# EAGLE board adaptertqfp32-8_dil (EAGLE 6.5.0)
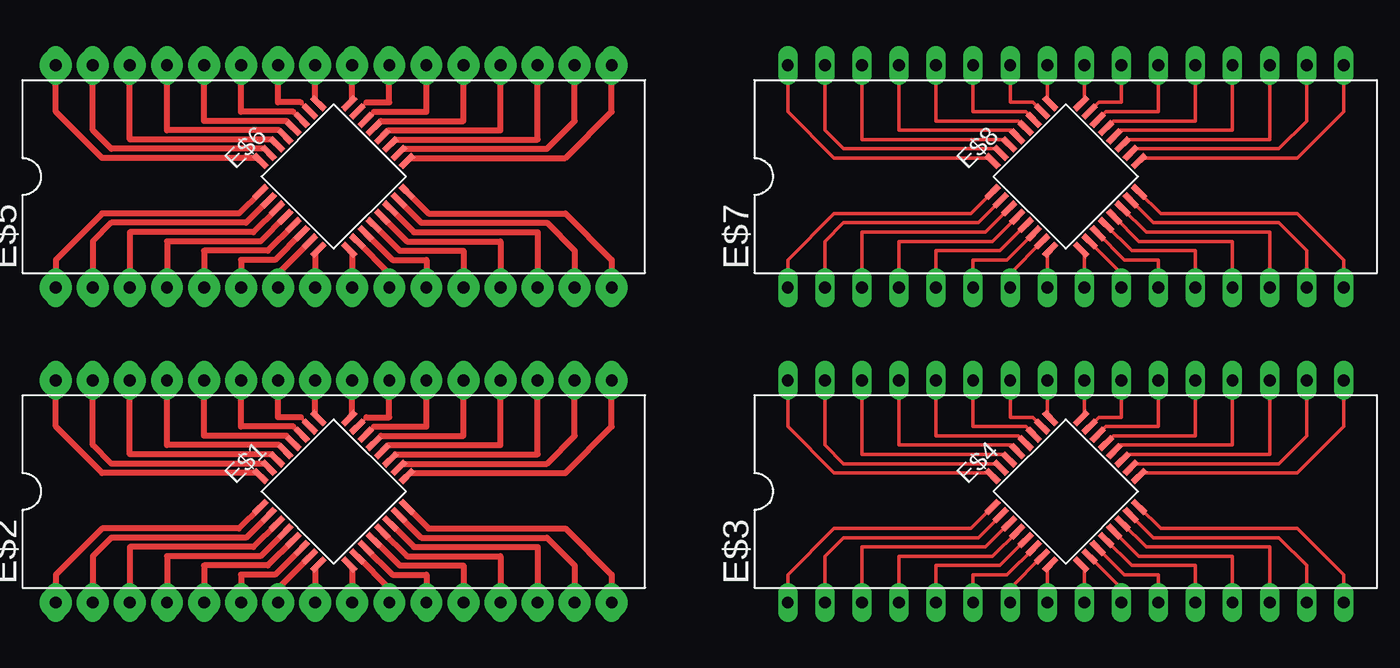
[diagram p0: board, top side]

No outline drawn. Coordinates in mm, seen from the top.
Copper layers (1*16): Top 0.035mm / dielectric 1.5mm / Bottom 0.035mm
Design rules "default": minimum track width 10mil, minimum drill 24mil, track to track 8mil, track to pad 8mil, pad to pad 8mil, via to via 8mil, smd to smd 8mil, copper to edge 40mil, drill to drill 8mil, minimum pad ring 10mil, minimum via ring 8mil, stop-mask expansion 4mil, vias tented up to drill 0mil, thermal gap 10mil

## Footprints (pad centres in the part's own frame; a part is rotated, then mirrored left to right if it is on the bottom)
LQFP32-7X7 = smd 1.2 x 0.4: 1 -4.3,2.8; 2 -4.3,2; 3 -4.3,1.2; 4 -4.3,0.4; 5 -4.3,-0.4; 6 -4.3,-1.2; 7 -4.3,-2; 8 -4.3,-2.8; 17 4.3,-2.8; 18 4.3,-2; 19 4.3,-1.2; 20 4.3,-0.4; 21 4.3,0.4; 22 4.3,1.2; 23 4.3,2; 24 4.3,2.8 | smd 0.4 x 1.2: 9 -2.8,-4.3; 10 -2,-4.3; 11 -1.2,-4.3; 12 -0.4,-4.3; 13 0.4,-4.3; 14 1.2,-4.3; 15 2,-4.3; 16 2.8,-4.3; 25 2.8,4.3; 26 2,4.3; 27 1.2,4.3; 28 0.4,4.3; 29 -0.4,4.3; 30 -1.2,4.3; 31 -2,4.3; 32 -2.8,4.3
DIL32 = drill 0.813 long: 1 -19.05,-7.62; 2 -16.51,-7.62; 3 -13.97,-7.62; 4 -11.43,-7.62; 5 -8.89,-7.62; 6 -6.35,-7.62; 7 -3.81,-7.62; 8 -1.27,-7.62; 9 1.27,-7.62; 10 3.81,-7.62; 11 6.35,-7.62; 12 8.89,-7.62; 13 11.43,-7.62; 14 13.97,-7.62; 15 16.51,-7.62; 16 19.05,-7.62; 17 19.05,7.62; 18 16.51,7.62; 19 13.97,7.62; 20 11.43,7.62; 21 8.89,7.62; 22 6.35,7.62; 23 3.81,7.62; 24 1.27,7.62; 25 -1.27,7.62; 26 -3.81,7.62; 27 -6.35,7.62; 28 -8.89,7.62; 29 -11.43,7.62; 30 -13.97,7.62; 31 -16.51,7.62; 32 -19.05,7.62

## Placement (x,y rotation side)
E$1  [LQFP32-7X7]  24.13,12.06 45 top
E$2  [DIL32]  24.13,12.06 0 top
E$3  [DIL32]  74.3,12.06 0 top
E$4  [LQFP32-7X7]  74.3,12.06 45 top
E$5  [DIL32]  24.13,33.66 0 top
E$6  [LQFP32-7X7]  24.13,33.66 45 top
E$7  [DIL32]  74.3,33.66 0 top
E$8  [LQFP32-7X7]  74.3,33.66 45 top

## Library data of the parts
E$1 E$4 E$6 E$8 = st-microelectronics
E$2 E$3 E$5 E$7 = atmel

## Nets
S$1: E$1.32 E$2.32
S$2: E$1.30 E$2.30
S$3: E$1.31 E$2.31
S$4: E$1.29 E$2.29
S$5: E$1.28 E$2.28
S$6: E$1.27 E$2.27
S$7: E$1.26 E$2.26
S$8: E$1.25 E$2.25
S$9: E$1.24 E$2.24
S$10: E$1.23 E$2.23
S$11: E$1.22 E$2.22
S$12: E$1.21 E$2.21
S$13: E$1.20 E$2.20
S$14: E$1.19 E$2.19
S$15: E$1.18 E$2.18
S$16: E$1.17 E$2.17
S$17: E$1.16 E$2.16
S$18: E$1.15 E$2.15
S$19: E$1.9 E$2.9
S$20: E$1.10 E$2.10
S$21: E$1.11 E$2.11
S$22: E$1.12 E$2.12
S$23: E$1.13 E$2.13
S$24: E$1.14 E$2.14
S$25: E$1.8 E$2.8
S$26: E$1.7 E$2.7
S$27: E$1.6 E$2.6
S$28: E$1.5 E$2.5
S$29: E$1.4 E$2.4
S$30: E$1.3 E$2.3
S$31: E$1.2 E$2.2
S$32: E$1.1 E$2.1
S$33: E$3.32 E$4.32
S$34: E$3.31 E$4.31
S$35: E$3.18 E$4.18
S$36: E$3.17 E$4.17
S$37: E$3.16 E$4.16
S$38: E$3.15 E$4.15
S$39: E$3.2 E$4.2
S$40: E$3.1 E$4.1
S$41: E$3.30 E$4.30
S$42: E$3.29 E$4.29
S$43: E$3.28 E$4.28
S$44: E$3.27 E$4.27
S$45: E$3.26 E$4.26
S$46: E$3.25 E$4.25
S$47: E$3.24 E$4.24
S$48: E$3.23 E$4.23
S$49: E$3.22 E$4.22
S$50: E$3.21 E$4.21
S$51: E$3.20 E$4.20
S$52: E$3.19 E$4.19
S$53: E$3.9 E$4.9
S$54: E$3.10 E$4.10
S$55: E$3.11 E$4.11
S$56: E$3.12 E$4.12
S$57: E$3.13 E$4.13
S$58: E$3.14 E$4.14
S$59: E$3.8 E$4.8
S$60: E$3.7 E$4.7
S$61: E$3.6 E$4.6
S$62: E$3.5 E$4.5
S$63: E$3.4 E$4.4
S$64: E$3.3 E$4.3
S$65: E$5.32 E$6.32
S$66: E$5.31 E$6.31
S$67: E$5.18 E$6.18
S$68: E$5.17 E$6.17
S$69: E$5.16 E$6.16
S$70: E$5.15 E$6.15
S$71: E$5.2 E$6.2
S$72: E$5.1 E$6.1
S$73: E$5.30 E$6.30
S$74: E$5.29 E$6.29
S$75: E$5.28 E$6.28
S$76: E$5.27 E$6.27
S$77: E$5.26 E$6.26
S$78: E$5.25 E$6.25
S$79: E$5.24 E$6.24
S$80: E$5.23 E$6.23
S$81: E$5.22 E$6.22
S$82: E$5.21 E$6.21
S$83: E$5.20 E$6.20
S$84: E$5.19 E$6.19
S$85: E$5.9 E$6.9
S$87: E$5.10 E$6.10
S$88: E$5.11 E$6.11
S$89: E$5.12 E$6.12
S$90: E$5.13 E$6.13
S$91: E$5.14 E$6.14
S$93: E$5.8 E$6.8
S$94: E$5.7 E$6.7
S$95: E$5.6 E$6.6
S$96: E$5.5 E$6.5
S$97: E$7.32 E$8.32
S$98: E$7.31 E$8.31
S$99: E$7.18 E$8.18
S$100: E$7.17 E$8.17
S$101: E$7.16 E$8.16
S$102: E$7.15 E$8.15
S$103: E$7.2 E$8.2
S$104: E$7.1 E$8.1
S$105: E$7.30 E$8.30
S$106: E$7.29 E$8.29
S$107: E$7.28 E$8.28
S$108: E$7.27 E$8.27
S$109: E$7.26 E$8.26
S$110: E$7.25 E$8.25
S$111: E$7.24 E$8.24
S$112: E$7.23 E$8.23
S$113: E$7.22 E$8.22
S$114: E$7.21 E$8.21
S$115: E$7.20 E$8.20
S$116: E$7.19 E$8.19
S$117: E$7.9 E$8.9
S$118: E$7.10 E$8.10
S$119: E$7.11 E$8.11
S$120: E$7.12 E$8.12
S$121: E$7.13 E$8.13
S$122: E$7.14 E$8.14
S$123: E$7.8 E$8.8
S$124: E$7.7 E$8.7
S$125: E$7.6 E$8.6
S$126: E$7.5 E$8.5
S$127: E$7.4 E$8.4
S$128: E$7.3 E$8.3
S$130: E$5.4 E$6.4
S$131: E$5.3 E$6.3

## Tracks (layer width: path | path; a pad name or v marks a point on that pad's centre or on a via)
S$1
  Top 0.254: E$1.32 18.9,13.34
  Top 0.406: E$2.32 5.08,16.51 8.26,13.34 18.9,13.34
S$2
  Top 0.254: E$1.30 19.89,14.61
  Top 0.406: 19.89,14.61 10.16,14.61 E$2.30
S$3
  Top 0.254: E$1.31 19.4,13.97
  Top 0.406: E$2.31 7.62,15.24 8.89,13.97 19.4,13.97
S$4
  Top 0.254: E$1.29 20.39,15.24
  Top 0.406: 20.39,15.24 12.7,15.24 E$2.29
S$5
  Top 0.254: E$1.28 20.89,15.88
  Top 0.406: 20.89,15.88 15.24,15.88 E$2.28
S$6
  Top 0.254: E$1.27 21.38,16.51
  Top 0.406: 21.38,16.51 17.78,16.51 E$2.27
S$7
  Top 0.254: E$1.26 21.88,17.14
  Top 0.406: 21.88,17.14 20.32,17.14 E$2.26
S$8
  Top 0.254: E$1.25 22.86,17.3
  Top 0.406: 22.86,17.3 E$2.25
S$9
  Top 0.254: E$1.24 25.4,17.3
  Top 0.406: 25.4,17.3 E$2.24
S$10
  Top 0.254: E$1.23 26.38,17.14
  Top 0.406: 26.38,17.14 27.94,17.14 E$2.23
S$11
  Top 0.254: E$1.22 26.88,16.51
  Top 0.406: 26.88,16.51 30.48,16.51 E$2.22
S$12
  Top 0.254: E$1.21 27.37,15.88
  Top 0.406: 27.37,15.88 33.02,15.88 E$2.21
S$13
  Top 0.254: E$1.20 27.87,15.24
  Top 0.406: 27.87,15.24 35.56,15.24 E$2.20
S$14
  Top 0.254: E$1.19 28.37,14.61
  Top 0.406: 28.37,14.61 38.1,14.61 E$2.19
S$15
  Top 0.254: E$1.18 28.86,13.97
  Top 0.406: E$2.18 40.64,15.88 38.73,13.97 28.86,13.97
S$16
  Top 0.254: E$1.17 29.36,13.34
  Top 0.406: E$2.17 43.18,16.51 40.01,13.34 29.36,13.34
S$17
  Top 0.406: E$2.16 43.18,6.35 40.01,9.53 30.63,9.53 E$1.16
S$18
  Top 0.406: E$2.15 40.64,6.99 38.73,8.89 30.13,8.89 E$1.15
S$19
  Top 0.254: E$1.9 25.4,6.83
  Top 0.406: 25.4,6.83 E$2.9
S$20
  Top 0.406: E$1.10 27.94,5.43 E$2.10
S$21
  Top 0.406: E$1.11 28.15,6.35 30.48,6.35 E$2.11
S$22
  Top 0.406: E$1.12 28.64,6.99 33.02,6.99 E$2.12
S$23
  Top 0.406: E$1.13 29.14,7.62 35.56,7.62 E$2.13
S$24
  Top 0.406: E$1.14 29.64,8.26 38.1,8.26 E$2.14
S$25
  Top 0.254: E$1.8 22.86,6.83
  Top 0.406: 22.86,6.83 E$2.8
S$26
  Top 0.406: E$1.7 20.32,5.43 E$2.7
S$27
  Top 0.406: E$1.6 20.11,6.35 17.78,6.35 E$2.6
S$28
  Top 0.406: E$1.5 19.62,6.99 15.24,6.99 E$2.5
S$29
  Top 0.406: E$1.4 19.12,7.62 12.7,7.62 E$2.4
S$30
  Top 0.406: E$1.3 18.62,8.26 10.16,8.26 E$2.3
S$31
  Top 0.406: E$2.2 7.62,7.62 8.89,8.89 18.13,8.89 E$1.2
S$32
  Top 0.406: E$2.1 5.08,6.35 8.26,9.53 17.63,9.53 E$1.1
S$33
  Top 0.254: E$3.32 55.24,16.51 58.42,13.34 69.06,13.34 E$4.32
S$34
  Top 0.254: E$3.31 57.78,15.24 59.05,13.97 69.56,13.97 E$4.31
S$35
  Top 0.254: E$3.18 90.81,15.88 88.9,13.97 79.03,13.97 E$4.18
S$36
  Top 0.254: E$3.17 93.34,16.51 90.17,13.34 79.53,13.34 E$4.17
S$37
  Top 0.254: E$3.16 93.34,6.35 90.17,9.53 80.8,9.53 E$4.16
S$38
  Top 0.254: E$3.15 90.81,6.99 88.9,8.89 80.3,8.89 E$4.15
S$39
  Top 0.254: E$3.2 57.78,7.62 59.05,8.89 68.29,8.89 E$4.2
S$40
  Top 0.254: E$3.1 55.24,6.35 58.42,9.53 67.8,9.53 E$4.1
S$41
  Top 0.254: E$4.30 70.06,14.61 60.33,14.61 E$3.30
S$42
  Top 0.254: E$4.29 70.55,15.24 62.87,15.24 E$3.29
S$43
  Top 0.254: E$4.28 71.05,15.88 65.41,15.88 E$3.28
S$44
  Top 0.254: E$4.27 71.55,16.51 67.94,16.51 E$3.27
S$45
  Top 0.254: E$4.26 72.04,17.14 70.48,17.14 E$3.26
S$46
  Top 0.254: E$4.25 73.03,17.3 E$3.25
S$47
  Top 0.254: E$4.24 75.56,17.3 E$3.24
S$48
  Top 0.254: E$4.23 76.55,17.14 78.11,17.14 E$3.23
S$49
  Top 0.254: E$4.22 77.04,16.51 80.64,16.51 E$3.22
S$50
  Top 0.254: E$4.21 77.54,15.88 83.19,15.88 E$3.21
S$51
  Top 0.254: E$4.20 78.04,15.24 85.72,15.24 E$3.20
S$52
  Top 0.254: E$4.19 78.53,14.61 88.27,14.61 E$3.19
S$53
  Top 0.254: E$4.9 75.56,6.83 E$3.9
S$54
  Top 0.254: E$4.10 78.11,5.43 E$3.10
S$55
  Top 0.254: E$4.11 78.31,6.35 80.64,6.35 E$3.11
S$56
  Top 0.254: E$4.12 78.81,6.99 83.19,6.99 E$3.12
S$57
  Top 0.254: E$4.13 79.31,7.62 85.72,7.62 E$3.13
S$58
  Top 0.254: E$4.14 79.8,8.26 88.27,8.26 E$3.14
S$59
  Top 0.254: E$4.8 73.03,6.83 E$3.8
S$60
  Top 0.254: E$4.7 70.48,5.43 E$3.7
S$61
  Top 0.254: E$4.6 70.28,6.35 67.94,6.35 E$3.6
S$62
  Top 0.254: E$4.5 69.78,6.99 65.41,6.99 E$3.5
S$63
  Top 0.254: E$4.4 69.28,7.62 62.87,7.62 E$3.4
S$64
  Top 0.254: E$4.3 68.79,8.26 60.33,8.26 E$3.3
S$65
  Top 0.254: E$6.32 18.9,34.92
  Top 0.406: E$5.32 5.08,38.1 8.26,34.92 18.9,34.92
S$66
  Top 0.254: E$6.31 19.4,35.56
  Top 0.406: E$5.31 7.62,36.83 8.89,35.56 19.4,35.56
S$67
  Top 0.254: E$6.18 28.86,35.56
  Top 0.406: E$5.18 40.64,37.47 38.73,35.56 28.86,35.56
S$68
  Top 0.254: E$6.17 29.36,34.92
  Top 0.406: E$5.17 43.18,38.1 40.01,34.92 29.36,34.92
S$69
  Top 0.406: E$5.16 43.18,27.94 40.01,31.11 30.63,31.11 E$6.16
S$70
  Top 0.406: E$5.15 40.64,28.57 38.73,30.48 30.13,30.48 E$6.15
S$71
  Top 0.406: E$5.2 7.62,29.21 8.89,30.48 18.13,30.48 E$6.2
S$72
  Top 0.406: E$5.1 5.08,27.94 8.26,31.11 17.63,31.11 E$6.1
S$73
  Top 0.254: E$6.30 19.89,36.2
  Top 0.406: 19.89,36.2 10.16,36.2 E$5.30
S$74
  Top 0.254: E$6.29 20.39,36.83
  Top 0.406: 20.39,36.83 12.7,36.83 E$5.29
S$75
  Top 0.254: E$6.28 20.89,37.47
  Top 0.406: 20.89,37.47 15.24,37.47 E$5.28
S$76
  Top 0.254: E$6.27 21.38,38.1
  Top 0.406: 21.38,38.1 17.78,38.1 E$5.27
S$77
  Top 0.254: E$6.26 21.88,38.73
  Top 0.406: 21.88,38.73 20.32,38.73 E$5.26
S$78
  Top 0.254: E$6.25 22.86,38.88
  Top 0.406: 22.86,38.88 E$5.25
S$79
  Top 0.254: E$6.24 25.4,38.88
  Top 0.406: 25.4,38.88 E$5.24
S$80
  Top 0.254: E$6.23 26.38,38.73
  Top 0.406: 26.38,38.73 27.94,38.73 E$5.23
S$81
  Top 0.254: E$6.22 26.88,38.1
  Top 0.406: 26.88,38.1 30.48,38.1 E$5.22
S$82
  Top 0.254: E$6.21 27.37,37.47
  Top 0.406: 27.37,37.47 33.02,37.47 E$5.21
S$83
  Top 0.254: E$6.20 27.87,36.83
  Top 0.406: 27.87,36.83 35.56,36.83 E$5.20
S$84
  Top 0.254: E$6.19 28.37,36.2
  Top 0.406: 28.37,36.2 38.1,36.2 E$5.19
S$85
  Top 0.254: E$6.9 25.4,28.43
  Top 0.406: 25.4,28.43 E$5.9
S$87
  Top 0.406: E$6.10 27.94,27.02 E$5.10
S$88
  Top 0.406: E$6.11 28.15,27.94 30.48,27.94 E$5.11
S$89
  Top 0.406: E$6.12 28.64,28.57 33.02,28.57 E$5.12
S$90
  Top 0.406: E$6.13 29.14,29.21 35.56,29.21 E$5.13
S$91
  Top 0.406: E$6.14 29.64,29.84 38.1,29.84 E$5.14
S$93
  Top 0.254: E$6.8 22.86,28.43
  Top 0.406: 22.86,28.43 E$5.8
S$94
  Top 0.406: E$6.7 20.32,27.02 E$5.7
S$95
  Top 0.406: E$6.6 20.11,27.94 17.78,27.94 E$5.6
S$96
  Top 0.406: E$6.5 19.62,28.57 15.24,28.57 E$5.5
S$97
  Top 0.254: E$7.32 55.24,38.1 58.42,34.92 69.06,34.92 E$8.32
S$98
  Top 0.254: E$7.31 57.78,36.83 59.05,35.56 69.56,35.56 E$8.31
S$99
  Top 0.254: E$7.18 90.81,37.47 88.9,35.56 79.03,35.56 E$8.18
S$100
  Top 0.254: E$7.17 93.34,38.1 90.17,34.92 79.53,34.92 E$8.17
S$101
  Top 0.254: E$7.16 93.34,27.94 90.17,31.11 80.8,31.11 E$8.16
S$102
  Top 0.254: E$7.15 90.81,28.57 88.9,30.48 80.3,30.48 E$8.15
S$103
  Top 0.254: E$7.2 57.78,29.21 59.05,30.48 68.29,30.48 E$8.2
S$104
  Top 0.254: E$7.1 55.24,27.94 58.42,31.11 67.8,31.11 E$8.1
S$105
  Top 0.254: E$8.30 70.06,36.2 60.33,36.2 E$7.30
S$106
  Top 0.254: E$8.29 70.55,36.83 62.87,36.83 E$7.29
S$107
  Top 0.254: E$8.28 71.05,37.47 65.41,37.47 E$7.28
S$108
  Top 0.254: E$8.27 71.55,38.1 67.94,38.1 E$7.27
S$109
  Top 0.254: E$8.26 72.04,38.73 70.48,38.73 E$7.26
S$110
  Top 0.254: E$8.25 73.03,38.88 E$7.25
S$111
  Top 0.254: E$8.24 75.56,38.88 E$7.24
S$112
  Top 0.254: E$8.23 76.55,38.73 78.11,38.73 E$7.23
S$113
  Top 0.254: E$8.22 77.04,38.1 80.64,38.1 E$7.22
S$114
  Top 0.254: E$8.21 77.54,37.47 83.19,37.47 E$7.21
S$115
  Top 0.254: E$8.20 78.04,36.83 85.72,36.83 E$7.20
S$116
  Top 0.254: E$8.19 78.53,36.2 88.27,36.2 E$7.19
S$117
  Top 0.254: E$8.9 75.56,28.43 E$7.9
S$118
  Top 0.254: E$8.10 78.11,27.02 E$7.10
S$119
  Top 0.254: E$8.11 78.31,27.94 80.64,27.94 E$7.11
S$120
  Top 0.254: E$8.12 78.81,28.57 83.19,28.57 E$7.12
S$121
  Top 0.254: E$8.13 79.31,29.21 85.72,29.21 E$7.13
S$122
  Top 0.254: E$8.14 79.8,29.84 88.27,29.84 E$7.14
S$123
  Top 0.254: E$8.8 73.03,28.43 E$7.8
S$124
  Top 0.254: E$8.7 70.48,27.02 E$7.7
S$125
  Top 0.254: E$8.6 70.28,27.94 67.94,27.94 E$7.6
S$126
  Top 0.254: E$8.5 69.78,28.57 65.41,28.57 E$7.5
S$127
  Top 0.254: E$8.4 69.28,29.21 62.87,29.21 E$7.4
S$128
  Top 0.254: E$8.3 68.79,29.84 60.33,29.84 E$7.3
S$129  (via drill 0.8 pad 2.18)
  other vias: 43.18,19.68 5.08,4.45 7.62,4.45 10.16,4.45 12.7,4.45 15.24,4.45 17.78,4.45 20.32,4.45 22.86,4.45 25.4,4.45 27.94,4.45 30.48,4.45 33.02,4.45 35.56,4.45 38.1,4.45 40.64,4.45 43.18,4.45 5.08,19.68 7.62,19.68 10.16,19.68 12.7,19.68 15.24,19.68 17.78,19.68 20.32,19.68 22.86,19.68 25.4,19.68 27.94,19.68 30.48,19.68 33.02,19.68 35.56,19.68 38.1,19.68 40.64,19.68
S$130
  Top 0.406: E$6.4 19.12,29.21 12.7,29.21 E$5.4
S$131
  Top 0.406: E$6.3 18.62,29.84 10.16,29.84 E$5.3
S$132  (via drill 0.8 pad 2.18)
  other vias: 43.18,41.27 5.08,26.04 7.62,26.04 10.16,26.04 12.7,26.04 15.24,26.04 17.78,26.04 20.32,26.04 22.86,26.04 25.4,26.04 27.94,26.04 30.48,26.04 33.02,26.04 35.56,26.04 38.1,26.04 40.64,26.04 43.18,26.04 5.08,41.27 7.62,41.27 10.16,41.27 12.7,41.27 15.24,41.27 17.78,41.27 20.32,41.27 22.86,41.27 25.4,41.27 27.94,41.27 30.48,41.27 33.02,41.27 35.56,41.27 38.1,41.27 40.64,41.27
